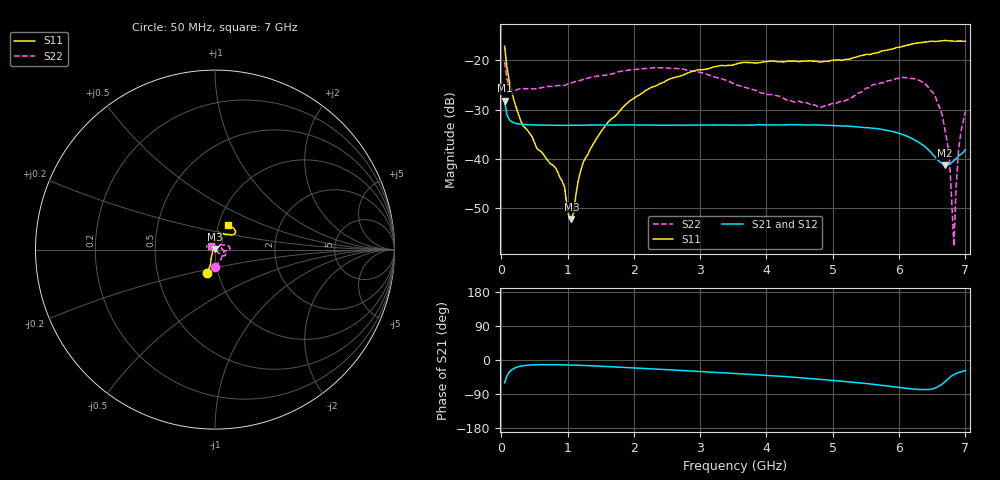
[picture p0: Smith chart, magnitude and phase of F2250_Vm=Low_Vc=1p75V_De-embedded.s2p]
! Integrated Device Technology
! Corporate Headquarters
! 6024 Silver Creek Valley Road
! San Jose, CA 95138  USA
! Phone:  1-408-284-8200
! Toll Free:  1-800-223-1366
! Webpage:  http://www.idt.com/
! Timing and RF Division
! 515 Groton Road, Suite 102
! Westford, MA 01886-6024
! Device:  F2250
! Description: Voltage Variable RF Attenuator
! Frequency:  50.0 -  6000.00 MHz
! Package:  3x3 mm Thin QFN Plastic Package: 16 pin
! Ports:  2 RF, 3 DC
!  Pin  1  = GND
!  Pin  2  = NC
!  Pin  3  = RF1  = Port 1
!  Pin  4  = NC
!  Pin  5  = GND
!  Pin  6  = GND
!  Pin  7  = GND
!  Pin  8  = GND
!  Pin  9  = NC
!  Pin 10  = RF2  = Port 2
!  Pin 11  = NC
!  Pin 12  = GND
!  Pin 13  = GND
!  Pin 14  = VCNTRL
!  Pin 15  = VDD
!  Pin 16  = VMODE
! Vcntrl:  1.750 Volts
! Vmode:  +0.000 Volts
! Vdd:  +3.30  Volts
! Current:  1.187 mA
! Data:  The device was measured on a the F2250 evaluation board which has
!  individual transmission lines to the RF pins.  Data was collected
!  using a calibrated network analyzer.  The evaluation board was
!  de-embedded using a TRL calibration technique.
!  The reference plane is the edge of the package pin.
! Misc:  SN 10
!  Action Tracker AT0258
! Date Measured:  2014-11-26
! Date:  2015-10-15  MJV
! Note:
!  Integrated Device Technology supplies this data as a sample of measured
!  data at the package pin for this product.  Your particular data for this
!  product may vary.
!  Data was taken at 25 degrees C.
!  Integrated Device Technology reserves the right to change this data at anytime.
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# GHz S dB R 50
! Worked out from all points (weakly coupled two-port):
!   201 points, 50 MHz to 7 GHz, reference 50 ohm
!   highest |S21| = -28.22 dB at 50 MHz (marker M1); lowest = -41.3 dB at 6.687 GHz (marker M2)
!   lowest |S11| = -52.2 dB at 1.058 GHz (marker M3), VSWR 1.00, Z = 49.9 + j0.225 ohm
!   |S11| at or under -10 dB: start of sweep to end of sweep
!   |S22| runs from -57.7 to -20.4 dB; largest |S21 - S12| = 9.5e-05
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0.05  -17.16 -108.2  -28.22 -60.1  -28.22 -60.1  -20.38 -88.6
0.1195  -24.20 -111.1  -32.02 -32.4  -32.03 -32.4  -25.35 -43.9
0.29325  -32.29 -126.3  -32.97 -16.3  -32.96 -16.3  -25.70 -18.0
0.84925  -42.63 170.7  -33.20 -12.5  -33.20 -12.5  -25.13 -7.3
0.9535  -45.68 170.6  -33.22 -12.8  -33.20 -12.8  -25.14 -7.0
1.023  -51.97 140.3  -33.18 -13.1  -33.19 -13.1  -24.73 -6.0
1.05775  -52.18 113.6  -33.19 -13.3  -33.19 -13.2  -24.61 -5.6
1.2315  -40.87 40.4  -33.18 -14.2  -33.16 -14.3  -23.90 -6.8
1.6485  -32.04 40.5  -33.13 -17.6  -33.14 -17.6  -22.86 -2.3
2.37825  -24.87 46.7  -33.14 -24.4  -33.13 -24.4  -21.54 5.5
3.525  -20.84 72.2  -33.16 -35.5  -33.17 -35.5  -24.89 26.1
4.7065  -20.22 72.2  -33.10 -49.6  -33.11 -49.6  -29.03 32.4
5.15825  -19.97 57.7  -33.36 -56.5  -33.35 -56.5  -28.33 8.9
5.85325  -17.84 40.3  -34.32 -69.2  -34.33 -69.2  -24.14 -21.2
6.40925  -16.33 41.7  -37.74 -78.1  -37.75 -78.1  -25.04 -37.0
6.54825  -16.21 45.0  -39.66 -73.5  -39.69 -73.4  -27.44 -41.5
6.68725  -16.01 48.7  -41.33 -58.1  -41.33 -57.8  -33.86 -41.7
6.75675  -16.08 51.0  -41.11 -47.5  -41.09 -47.5  -39.19 -44.8
6.82625  -16.16 53.4  -40.35 -38.6  -40.30 -38.6  -57.68 175.4
6.861  -16.15 55.0  -39.95 -35.6  -39.92 -35.7  -45.45 143.0
6.89575  -16.12 56.9  -39.42 -33.3  -39.37 -33.4  -38.50 131.5
7  -16.15 63.1  -38.14 -27.7  -38.12 -27.6  -30.39 135.0
